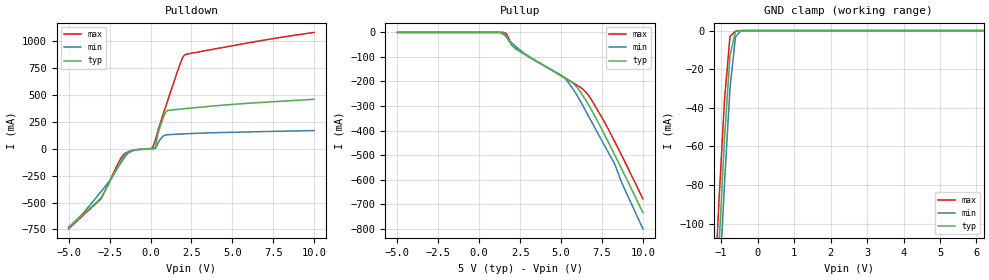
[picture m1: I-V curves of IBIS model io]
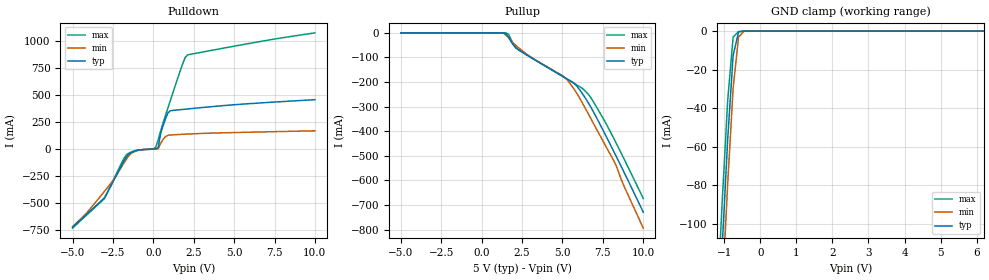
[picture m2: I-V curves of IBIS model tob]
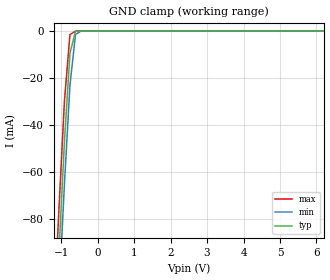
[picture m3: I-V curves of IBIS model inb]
|   TEXAS INSTRUMENTS INCORPORATED
|   Advanced Bus Interface Group
|   IBIS Model of ABT18502
|   18-bit Registered Bus Transceivers
|   64-pin PM Package
[IBIS Ver]   2.1
[File name]   abt18502.ibs
[File Rev]   1.6   | from silicon model only
[Date]   97215
[Source]   Silicon-level SPICE model at Texas Instruments (ALEY)
[Notes]   The following is an IBIS list for the ABT18502.
|   - SCAN TEST DEVICES WITH 18-BIT UNIVERSAL BUS TRANSCEIVERS
   !! SN74ABTH18502A is available and preferred vs SN74ABT18502 !!
   - This file may be incomplete or may not be fully compliant
   with the IBIS specification. It will be replaced with a
   version that is IBIS Revision 3.2 compliant and is complete
   and accurate.  Please email all questions and comments to
   sllibis@ti.com.
   Release 1.5) 97100 ALEY - initial release
   Release 1.6) 97215 ALEY - fixed load for ramp (rising) measurement
   includes all available commercial packages:
   PM=64TQFP (no-coupling model)
[Disclaimer]
   Property of Texas Instruments Incorporated.  Unauthorized
   reproduction and/or distribution is strictly prohibited.
   This product is protected under copyright law.
   Created 1997, (C) Copyright 1997, Texas Instruments Incorporated.
   All Rights Reserved
   UNLESS THERE IS A SIGNED, WRITTEN AGREEMENT TO THE
   CONTRARY, TEXAS INSTRUMENTS ("TI") IS PROVIDING THE IBIS
   MODELS "AS IS" AND WITHOUT ANY WARRANTY, EXPRESSED OR
   IMPLIED.  TI assumes no liability for:
   1) the accuracy of the IBIS models provided to your
   company;
   2) the proper functioning of these IBIS models in your
   design or for any resulting applications; or
   3) infringement of patents, copyrights or intellectual
   property rights resulting from your use of these IBIS
   models.
   TI provides IBIS Models as a service to our customers.
   You and your company shall not distribute, sell or give
   these models to anyone else without prior written
   permission from TI.
   TI reserves the right to make changes to our products or
   to discontinue any semiconductor product or service
   without notice, and advises our customers to obtain the
   latest version of relevant information to verify, before
   placing orders, that the information being relied on is
   current.
   Please be aware that your receipt and use of the IBIS
   information provided shall serve as acceptance of these
   terms and conditions.  If you do not accept these terms,
   you should return or destroy the IBIS models and any
   other accompanying information immediately.
[Component]   SN74ABT18502_PM
[Manufacturer]  Texas Instruments
[Package]
|   typ   min   max
R_pkg   0.079   0.069   0.101
L_pkg   3.757nH   1.665nH   4.658nH
C_pkg   0.134pF   0.017pF   0.289pF
[Pin]   signal_name   model_name   R_pin   L_pin   C_pin
1   1A3   io   0.085   4.537nH   0.271pF
2   1A4   io   0.085   4.357nH   0.165pF
3   1A5   io   0.085   4.193nH   0.139pF
4   GND   GND   0.085   4.094nH   0.14pF
5   1A6   io   0.085   3.956nH   0.116pF
6   1A7   io   0.085   3.858nH   0.108pF
7   1A8   io   0.084   3.77nH   0.102pF
8   1A9   io   0.085   3.744nH   0.103pF
9   VCC   POWER   0.085   3.738nH   0.099pF
10   2A1   io   0.085   3.778nH   0.101pF
11   2A2   io   0.085   3.837nH   0.106pF
12   2A3   io   0.085   3.935nH   0.115pF
13   GND   GND   0.085   4.08nH   0.14pF
14   2A4   io   0.086   4.193nH   0.139pF
15   2A5   io   0.085   4.302nH   0.162pF
16   2A6   io   0.085   4.492nH   0.269pF
17   2A7   io   0.087   4.341nH   0.275pF
18   2A8   io   0.07   3.792nH   0.153pF
19   2A9   io   0.071   3.671nH   0.129pF
20   GND   GND   0.071   3.581nH   0.131pF
21   2OEAB_BAR   inb   0.07   3.48nH   0.112pF
22   2LEAB   inb   0.07   3.469nH   0.107pF
23   2CLKAB   inb   0.071   3.424nH   0.099pF
24   TDI   inu   0.071   3.408nH   0.101pF
25   VCC   POWER   0.07   3.428nH   0.099pF
26   TCK   inb   0.07   3.439nH   0.098pF
27   2CLKBA   inb   0.072   3.551nH   0.107pF
28   2LEBA   inb   0.07   3.63nH   0.12pF
29   GND   GND   0.071   3.597nH   0.136pF
30   2OEBA_BAR   inb   0.071   3.685nH   0.13pF
31   2B9   io   0.071   3.797nH   0.153pF
32   2B8   io   0.089   4.378nH   0.277pF
33   2B7   io   0.085   4.496nH   0.27pF
34   2B6   io   0.085   4.31nH   0.162pF
35   2B5   io   0.086   4.189nH   0.138pF
36   GND   GND   0.086   4.084nH   0.139pF
37   2B4   io   0.085   3.942nH   0.115pF
38   2B3   io   0.085   3.843nH   0.104pF
39   2B2   io   0.085   3.824nH   0.103pF
40   2B1   io   0.086   3.832nH   0.107pF
41   VCC   POWER   0.085   3.837nH   0.103pF
42   1B9   io   0.086   3.846nH   0.102pF
43   1B8   io   0.086   3.886nH   0.104pF
44   1B7   io   0.085   3.971nH   0.115pF
45   GND   GND   0.085   4.131nH   0.14pF
46   1B6   io   0.085   4.26nH   0.139pF
47   1B5   io   0.085   4.413nH   0.163pF
48   1B4   io   0.085   4.632nH   0.273pF
49   1B3   io   0.101   4.658nH   0.289pF
50   1B2   io   0.084   4.025nH   0.164pF
51   1B1   io   0.071   3.636nH   0.129pF
52   GND   GND   0.072   3.566nH   0.132pF
53   1OEBA_BAR   inb   0.071   3.482nH   0.112pF
54   1LEBA   inb   0.071   3.452nH   0.107pF
55   1CLKBA   inb   0.071   3.413nH   0.102pF
56   TMS   inu   0.072   3.488nH   0.112pF
57   VCC   POWER   0.072   3.487nH   0.106pF
58   TDO   tob   0.071   3.412nH   0.099pF
59   1CLKAB   inb   0.071   3.449nH   0.104pF
60   1LEAB   inb   0.07   3.505nH   0.113pF
61   GND   GND   0.071   3.6nH   0.134pF
62   1OEAB_BAR   inb   0.071   3.678nH   0.131pF
63   1A1   io   0.071   3.838nH   0.156pF
64   1A2   io   0.089   4.4nH   0.278pF
| Models and submodels in the file (4): io (I/O), tob (3-state), inb (Input), inu (Input)
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[Model]   io
| high-drive I/O buffer
| inb18502.abt (95265 SRIJ)
| tob18502.abt (95265 SRIJ)
| pad18502.abt (95265 SRIJ)
Model_type   I/O
Polarity   Non-Inverting
| Signals   1A1..2A9, 1B1..2B9
Vinl = 0.8V
Vinh = 2.0V
| variable   typ   min   max
C_comp   11pF   NA   NA
| variable   typ   min   max
[Voltage range]   5.0V   4.5V   5.5V
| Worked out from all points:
|   slope of the pulldown table from 0 to 0.75 V, typ, clamps not added: 2.68 ohm
|   GND clamp passes 1 mA (typ) near -0.61 V on its own axis
[pullup]
|   50C:5V:   100C:4.5V:weak   0C:5.5V:strong
|   Voltage   I(typ)   I(min)   I(max)
-5V       8.889nA    9.085nA    9.096nA
1.061V    -1.634uA   -30.97uA   -28.12nA
1.515V    -3.937mA   -9.82mA    -394.6uA
1.667V    -17.91mA   -20.21mA   -6.057mA
2.121V    -61.04mA   -51.08mA   -61.24mA
5.152V    -182.1mA   -181.8mA   -182.7mA
5.909V    -218.5mA   -248.8mA   -212.5mA
6.364V    -260.8mA   -302.1mA   -233.6mA
6.818V    -310.6mA   -358mA     -270.6mA
8.182V    -486mA     -524mA     -432.3mA
8.788V    -567.5mA   -624.1mA   -512.6mA
10V       -734.6mA   -800.1mA   -678.1mA
[pulldown]
|   50C:5V:   100C:4.5V:weak   0C:5.5V:strong
|   Voltage   I(typ)   I(min)   I(max)
-5V       -734.3mA   -727.7mA   -742.3mA
-4.091V   -606mA     -593.7mA   -613.8mA
-3.03V    -456.4mA   -398.8mA   -464.8mA
-1.667V   -74.92mA   -95.9mA    -55.84mA
-1.061V   -15.58mA   -19.71mA   -13.59mA
151.5mV   71.79uA    217.1uA    17.24mA
303mV     15.38mA    1.979mA    86.75mA
454.5mV   145.9mA    51.8mA     169.4mA
909.1mV   336.7mA    127mA      384.9mA
1.818V    367.6mA    136.1mA    792.7mA
2.121V    372.1mA    138.4mA    875mA
10V       458.6mA    168.6mA    1.08A
[gnd_clamp]
|   50C:5V:   100C:4.5V:weak   0C:5.5V:strong
|   Voltage   I(typ)   I(min)   I(max)
-5V       -2.206A    -2.215A    -2.196A
-1.212V   -172mA     -197.3mA   -146.7mA
-1.061V   -112.1mA   -136.8mA   -88.59mA
-909.1mV  -56.46mA   -79.59mA   -36.18mA
-757.6mV  -12.77mA   -29.77mA   -3.031mA
-606.1mV  -427.8uA   -3.106mA   -239uA
-454.5mV  -3.122uA   -95.22uA   -14.93uA
-303mV    -67.92nA   -1.085uA   -80.05nA
10V       9.609nA    10.07nA    9.584nA
[ramp]
| variable   typ   min   max
dV/dt_r   1.7346E+00/7.1499E-10  1.4463E+00/1.0357E-09  1.9515E+00/5.5277E-10
dV/dt_f   2.7863E+00/2.0056E-09  2.3647E+00/2.9438E-09  3.1042E+00/1.3742E-09
[Model]   tob
| three-state output buffer
| tob18502.abt (95265 SRIJ)
| pad18502.abt (95265 SRIJ)
Model_type   3-state
Polarity   Non-Inverting
| Signals   TDO
| variable   typ   min   max
C_comp   5pF   NA   NA
| variable   typ   min   max
[Voltage range]   5.0V   4.5V   5.5V
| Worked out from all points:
|   slope of the pulldown table from 0 to 0.75 V, typ, clamps not added: 2.68 ohm
|   GND clamp passes 1 mA (typ) near -0.61 V on its own axis
[pullup]
|   50C:5V:   100C:4.5V:weak   0C:5.5V:strong
|   Voltage   I(typ)   I(min)   I(max)
-5V       7.89nA     8.134nA    8.046nA
1.061V    -1.634uA   -30.97uA   -28.57nA
1.515V    -3.937mA   -9.82mA    -394.6uA
1.667V    -17.91mA   -20.21mA   -6.057mA
2.121V    -61.04mA   -51.08mA   -61.24mA
5.152V    -182.1mA   -181.7mA   -182.7mA
5.909V    -218.2mA   -248mA     -212.5mA
6.364V    -260.1mA   -300.8mA   -233.5mA
6.818V    -309.4mA   -356.2mA   -270mA
8.182V    -483.2mA   -520.4mA   -430.1mA
8.788V    -563.9mA   -619.7mA   -509.7mA
10V       -729.4mA   -794.1mA   -673.6mA
[pulldown]
|   50C:5V:   100C:4.5V:weak   0C:5.5V:strong
|   Voltage   I(typ)   I(min)   I(max)
-5V       -729.1mA   -722.4mA   -737.1mA
-4.091V   -602mA     -589.6mA   -609.8mA
-3.03V    -453.8mA   -396.1mA   -462.2mA
-1.667V   -73.9mA    -94.79mA   -54.89mA
-1.061V   -15.21mA   -19.26mA   -13.29mA
151.5mV   71.79uA    217.1uA    17.24mA
303mV     15.38mA    1.979mA    86.75mA
454.5mV   145.9mA    51.8mA     169.4mA
909.1mV   336.7mA    127mA      384.9mA
1.818V    367.6mA    136.1mA    792.7mA
2.121V    372.1mA    138.4mA    875mA
10V       458.6mA    168.6mA    1.08A
[gnd_clamp]
|   50C:5V:   100C:4.5V:weak   0C:5.5V:strong
|   Voltage   I(typ)   I(min)   I(max)
-5V       -2.2A      -2.21A     -2.191A
-1.212V   -171.5mA   -196.7mA   -146.2mA
-1.061V   -111.7mA   -136.4mA   -88.3mA
-909.1mV  -56.25mA   -79.3mA    -36.04mA
-757.6mV  -12.69mA   -29.62mA   -3.007mA
-606.1mV  -423.5uA   -3.071mA   -238.9uA
-454.5mV  -3.099uA   -94.4uA    -14.93uA
-303mV    -67.78nA   -1.077uA   -80.02nA
10V       8.609nA    9.067nA    8.584nA
[ramp]
| variable   typ   min   max
dV/dt_r   1.7348E+00/6.9978E-10  1.4466E+00/1.0194E-09  1.9518E+00/5.6447E-10
dV/dt_f   2.7864E+00/2.0064E-09  2.3649E+00/2.9298E-09  3.1043E+00/1.3836E-09
[Model]   inb
| high-impedance input buffer
| inb18502.abt (95265 SRIJ)
| pad18502.abt (95265 SRIJ)
Model_type   Input
Polarity   Non-Inverting
| Signals   CLK, LE, OE#, TCK
Vinl = 0.8V
Vinh = 2.0V
| variable   typ   min   max
C_comp   5pF   NA   NA
| variable   typ   min   max
[Voltage range]   5.0V   4.5V   5.5V
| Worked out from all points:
|   GND clamp passes 1 mA (typ) near -0.62 V on its own axis
[gnd_clamp]
|   50C:5V:   100C:4.5V:weak   0C:5.5V:strong
|   Voltage   I(typ)   I(min)   I(max)
-5V       -1.478A    -1.494A    -1.462A
-1.212V   -144.3mA   -162.8mA   -125.9mA
-1.061V   -94.32mA   -112.9mA   -76.01mA
-909.1mV  -47.12mA   -65.07mA   -29.8mA
-757.6mV  -9.358mA   -23.03mA   -1.482mA
-606.1mV  -116.2uA   -1.455mA   -3.299uA
-454.5mV  -577nA     -16.82uA   -6.183nA
10V       2nA        2.017nA    2nA
